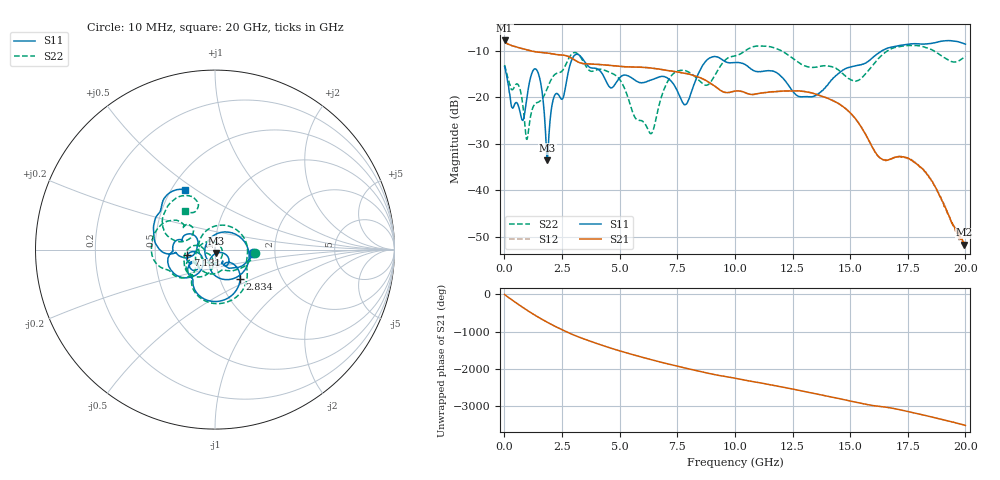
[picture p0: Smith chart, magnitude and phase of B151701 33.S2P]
!  2-Port S-parameters saved by WinCal
! VAR MeasName=S-Parameters (CALIBRATED_DATA) read from VNA (N5244A)
! VAR MeasDate=2015-12-24 19:13:12
! VAR NAME=B151701 33
! VAR FILENAME=B151701 33.S2P
! VAR DATE=2015-12-24 19:13:12
! VAR PHYS_PORTS=1,3
# Hz S DB R 50
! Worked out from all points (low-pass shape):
!   801 points, 10 MHz to 20 GHz, reference 50 ohm
!   highest |S21| = -7.82 dB at 10 MHz (marker M1); lowest = -51.8 dB at 19.95 GHz (marker M2)
!   |S21| within 3 dB of the highest: start of sweep to 2.224 GHz
!   lowest |S11| = -33.6 dB at 1.859 GHz (marker M3), VSWR 1.04, Z = 50.7 - j1.97 ohm
!   |S11| at or under -10 dB: start of sweep to 16.39 GHz
!   |S22| runs from -29.1 to -8.9 dB; largest |S21 - S12| = 0.0016
!   S11 on the Smith chart (normalised r, x): 10 MHz: 1.54, -0.06; 2.834 GHz: 1.24, -0.43; 7.131 GHz: 0.73, -0.05; 20 GHz: 0.59, +0.45
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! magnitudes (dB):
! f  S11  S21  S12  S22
! 10 MHz  -13.4  -7.8  -7.8  -13.1
! 759.6 MHz  -24.8  -9.6  -9.5  -20.3
! 984.5 MHz  -19.8  -9.8  -9.8  -29.1
! 1.434 GHz  -14.4  -10.3  -10.3  -21.2
! 1.859 GHz  -33.6  -10.5  -10.5  -18.2
! 2.134 GHz  -20.3  -10.7  -10.7  -15.4
! 2.534 GHz  -20.3  -11.0  -11.0  -14.2
! 2.834 GHz  -13.3  -11.4  -11.4  -11.3
! 3.358 GHz  -11.5  -12.7  -12.7  -11.8
! 4.933 GHz  -16.3  -13.3  -13.3  -15.8
! 6.332 GHz  -16.4  -13.7  -13.7  -27.8
! 6.682 GHz  -15.7  -14.0  -14.0  -22.3
! 7.131 GHz  -16.1  -14.3  -14.3  -16.2
! 7.856 GHz  -21.6  -14.9  -14.9  -14.3
! 8.806 GHz  -11.9  -16.6  -16.6  -17.4
! 10.01 GHz  -12.6  -18.7  -18.7  -11.1
! 13.35 GHz  -19.9  -19.1  -19.1  -13.6
! 15.3 GHz  -13.2  -25.1  -25.1  -16.5
! 16.68 GHz  -9.4  -33.5  -33.4  -9.9
! 18.25 GHz  -8.6  -36.1  -36.1  -9.3
! 19.95 GHz  -8.5  -51.8  -51.3  -11.4
! 20 GHz  -8.6  -51.8  -52.0  -11.2
